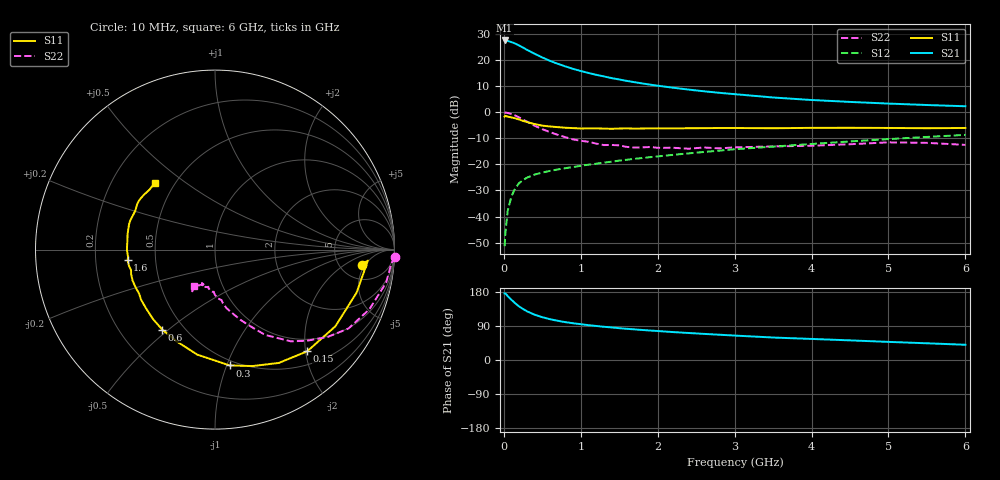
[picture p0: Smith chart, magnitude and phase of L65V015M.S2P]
!  INFINEON TECHNOLOGIES Small Signal Semiconductors
! BFR380L3 , Si-NPN RF-Transistor in TSLP-3-1
!  Vce=5 V,  Ic=15 mA
! Common Emitter S-Parameters:  07. March 2005
#  GHz  S  MA  R  50
! f  S11  S21  S12  S22
! GHz  Mag  Ang  Mag  Ang  Mag  Ang  Mag  Ang
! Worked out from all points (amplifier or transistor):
!   36 points, 10 MHz to 6 GHz, reference 50 ohm
!   highest |S21| = 27.6 dB at 10 MHz (marker M1)
!   |S21| within 3 dB of that: start of sweep to 265.3 MHz
!   unconditionally stable (mu >= 1): 2.325 GHz to 4.677 GHz
!   at 250 MHz: K = 0.26, MSG = 25.4 dB, |S12| = -26.0 dB
!   at 1.4 GHz: K = 0.88, MSG = 16.0 dB, |S12| = -19.0 dB
!   at 6 GHz: K = 0.96, MSG = 5.5 dB, |S12| = -8.7 dB
!   S11 on the Smith chart (normalised r, x): 10 MHz: 8.10, -4.16; 150 MHz: 0.74, -2.03; 300 MHz: 0.46, -1.02; 600 MHz: 0.38, -0.48; 1.6 GHz: 0.34, -0.05; 6 GHz: 0.39, +0.38
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0.01  0.8225 -5.8  23.87 175.8  0.0027 78.9  1.003 -2.2
0.02  0.854 -4.1  23.81 175.6  0.0048 92.2  0.9855 -4.5
0.05  0.8246 -16.9  23.35 168.8  0.0129 82.2  0.9713 -10.9
0.1  0.7953 -32.5  22.18 158.7  0.0247 75.1  0.9223 -21.1
0.15  0.7649 -47.8  20.75 149.2  0.0352 68.3  0.864 -30.6
0.2  0.7247 -60.6  19.04 141.1  0.044 63.3  0.7948 -37.7
0.25  0.6819 -72.1  17.4 134.5  0.0499 59.2  0.7209 -44.8
0.3  0.6505 -82.8  15.81 128.6  0.0557 55.8  0.6633 -50.4
0.4  0.5933 -99.6  13.26 119.5  0.0638 51.9  0.5523 -59.5
0.5  0.5545 -112.5  11.27 113.0  0.0698 50.4  0.4741 -64.9
0.6  0.5338 -123.4  9.692 107.6  0.0751 49.5  0.4162 -70.1
0.7  0.519 -131.6  8.521 103.5  0.08 49.9  0.3694 -74.5
0.8  0.5051 -139.3  7.582 99.9  0.0846 50.2  0.3333 -78.8
1.1  0.4897 -155.1  5.678 91.9  0.0989 52.2  0.2717 -86.9
1.4  0.4815 -166.1  4.533 86.0  0.1128 54.4  0.2361 -92.9
1.6  0.4907 -173.1  3.997 82.3  0.1231 55.3  0.2164 -99.9
2.2  0.4907 174.1  2.959 73.7  0.1525 58.3  0.2087 -105.5
2.8  0.4993 163.4  2.365 66.7  0.1834 60.1  0.2029 -113.4
3.5  0.4941 153.8  1.922 59.3  0.2194 59.8  0.2215 -115.4
4.5  0.5038 146.6  1.58 51.8  0.2759 60.2  0.2438 -117.5
5.5  0.4947 137.7  1.378 44.1  0.3365 58.0  0.2591 -118.8
6  0.5 132.3  1.305 40.2  0.3687 56.4  0.2367 -119.8
